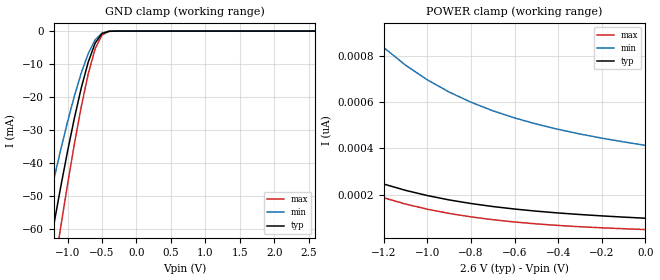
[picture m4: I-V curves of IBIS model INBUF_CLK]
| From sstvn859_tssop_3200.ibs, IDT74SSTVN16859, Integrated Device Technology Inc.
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|   Model INBUF_CLK
[Model]   INBUF_CLK
Model_type   Input
Polarity   Non-Inverting
Vinl =  0.79000V
Vinh =  1.71000V
C_comp   3.28000pF   3.28000pF   3.28000pF
[Temperature Range]   25.00000   70.00000   0.000
[Voltage Range]   2.60000V   2.50000V   2.70000V
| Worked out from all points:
|   GND clamp passes 1 mA (typ) near -0.51 V on its own axis
[GND_clamp]
| voltage   I(typ)   I(min)   I(max)
-2.6V     -234.1mA   -191.2mA   -271.3mA
-1.4V     -82.75mA   -64.31mA   -101.1mA
-1.3V     -70.61mA   -54.52mA   -86.97mA
-1.2V     -58.76mA   -45.05mA   -73.07mA
-1.1V     -47.31mA   -35.99mA   -59.51mA
-900mV    -26.27mA   -19.6mA    -34.1mA
-800mV    -17.12mA   -12.63mA   -22.79mA
-700mV    -9.383mA   -6.816mA   -12.96mA
-600mV    -3.667mA   -2.639mA   -5.378mA
-500mV    -745.8uA   -564.9uA   -1.16mA
-300mV    -3.071uA   -4.017uA   -3.937uA
2.6V      98.92pA    428.4pA    47.06pA
[POWER_clamp]
| voltage   I(typ)   I(min)   I(max)
-2.6V     1.876nA    5.37nA     1.896nA
-2.2V     1.035nA    3.042nA    1.003nA
-2.1V     889.8pA    2.636nA    850.6pA
-2V       764.4pA    2.286nA    719.6pA
-1.9V     656.9pA    1.985nA    607.8pA
-1.7V     487pA      1.509nA    432.1pA
-1.5V     365.1pA    1.168nA    307.2pA
-1.3V     279.1pA    927.1pA    219.9pA
-1V       196.7pA    696.1pA    137.8pA
-800mV    162.4pA    599.6pA    104.7pA
-500mV    129.4pA    505.4pA    74.46pA
0V        98.92pA    413.5pA    50.07pA
